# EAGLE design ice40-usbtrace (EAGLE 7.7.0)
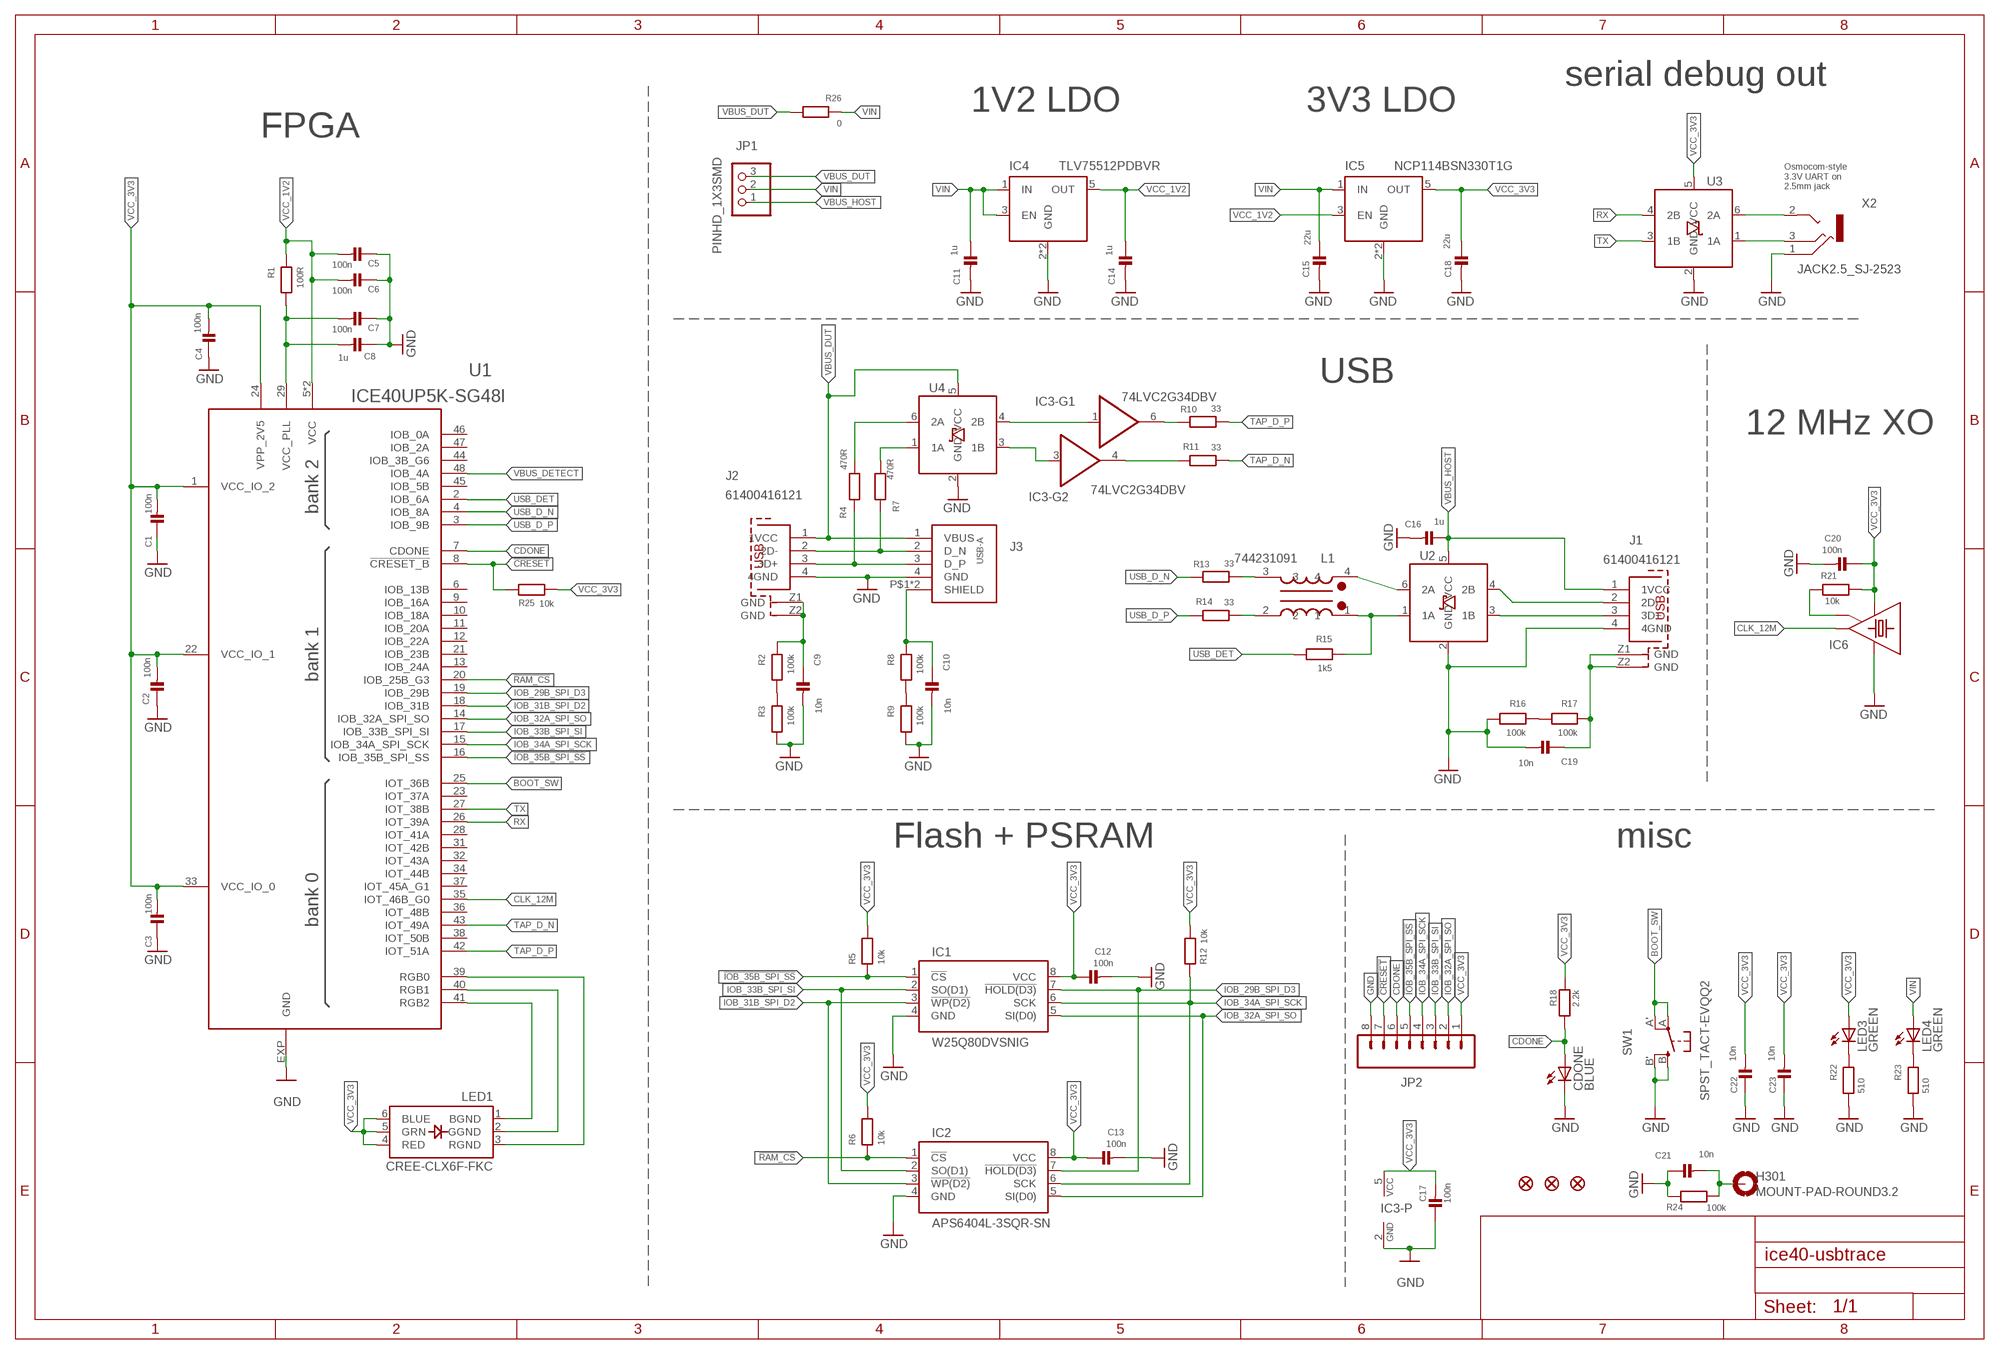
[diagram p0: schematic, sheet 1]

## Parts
C1  100n  CAP_CERAMIC_0603  [_0603]
C2  100n  CAP_CERAMIC_0603  [_0603]
C3  100n  CAP_CERAMIC_0603  [_0603]
C4  100n  CAP_CERAMIC_0603  [_0603]
C5  100n  CAP_CERAMIC_0603  [_0603]
C6  100n  CAP_CERAMIC_0603  [_0603]
C7  100n  CAP_CERAMIC_0603  [_0603]
C8  1u  CAP_CERAMIC_0603  [_0603]
C9  10n  CAP_CERAMIC_0402  [_0402]
C10  10n  CAP_CERAMIC_0402  [_0402]
C11  1u  CAP_CERAMIC_0603  [_0603]
C12  100n  CAP_CERAMIC_0603  [_0603]
C13  100n  CAP_CERAMIC_0603  [_0603]
C14  1u  CAP_CERAMIC_0603  [_0603]
C15  22u  CAP_CERAMIC1206  [1206]
C16  1u  CAP_CERAMIC_0603  [_0603]
C17  100n  CAP_CERAMIC_0603  [_0603]
C18  22u  CAP_CERAMIC1206  [1206]
C19  10n  CAP_CERAMIC_0402  [_0402]
C20  100n  CAP_CERAMIC_0603  [_0603]
C21  10n  CAP_CERAMIC_0402  [_0402]
C22  10n  CAP_CERAMIC_0402  [_0402]
C23  10n  CAP_CERAMIC_0402  [_0402]
CDONE  BLUE  LEDCHIPLED_0603  [CHIPLED_0603]
FID1  FIDUCIAL""  [FIDUCIAL_1MM]
FID2  FIDUCIAL""  [FIDUCIAL_1MM]
FID3  FIDUCIAL""  [FIDUCIAL_1MM]
H301  MOUNT-PAD-ROUND3.2  [3,2-PAD]
IC1  W25Q80DVSNIG  AT25SF-COMB  [SO08COMBINED]
IC2  APS6404L-3SQR-SN  AT25SF-COMB  [SO08COMBINED]
IC3  74LVC2G34DBV  [DBV_R-PDSO-G6]
IC4  TLV75512PDBVR  TLV70033-SOT  [SOT23-DBV]
IC5  NCP114BSN330T1G  TLV70033-SOT  [SOT23-DBV]
IC6  OSCILLATOR-4-SMD-2X2.5MM  [CRYSTAL-SMD-2X2.5MM]
J1  61400416121  [61400416121]
J2  61400416121  [61400416121]
J3  USB-A-HORIZ  [USB_A_HORIZ]
JP1  PINHD_1X3SMD  [1X03_SMD]
JP2  M08LOCK  [1X08_LOCK]
L1  744231091  WE-CNSW_0805  [WE-CNSW_0805]
LED1  CREE-CLX6F-FKC  [CREE-CLX6F-FKC_PLCC6]
LED3  GREEN  LEDCHIP-LED0603  [CHIP-LED0603]
LED4  GREEN  LEDCHIP-LED0603  [CHIP-LED0603]
R1  100R  RESISTOR_0603  [_0603]
R2  100k  RESISTOR_0603  [_0603]
R3  100k  RESISTOR_0603  [_0603]
R4  470R  RESISTOR_0603  [_0603]
R5  10k  RESISTOR_0603  [_0603]
R6  10k  RESISTOR_0603  [_0603]
R7  470R  RESISTOR_0603  [_0603]
R8  100k  RESISTOR_0603  [_0603]
R9  100k  RESISTOR_0603  [_0603]
R10  33  RESISTOR_0402  [_0402]
R11  33  RESISTOR_0402  [_0402]
R12  10k  RESISTOR_0603  [_0603]
R13  33  RESISTOR_0402  [_0402]
R14  33  RESISTOR_0402  [_0402]
R15  1k5  RESISTOR_0603  [_0603]
R16  100k  RESISTOR_0603  [_0603]
R17  100k  RESISTOR_0603  [_0603]
R18  2.2k  RESISTOR_0603  [_0603]
R21  10k  RESISTOR_0603  [_0603]
R22  510  RESISTOR_0603  [_0603]
R23  510  RESISTOR_0603  [_0603]
R24  100k  RESISTOR_0603  [_0603]
R25  10k  RESISTOR_0603  [_0603]
R26  0  RESISTOR_0603  [_0603]
SW1  SPST_TACT-EVQQ2  [EVQ-Q2]
U1  ICE40UP5K-SG48I  [QFN48]
U2  IP4234CZ6  [TSOP-6]
U3  IP4234CZ6  [TSOP-6]
U4  IP4234CZ6  [TSOP-6]
X2  JACK2.5_SJ-2523  [JACK2.5_SJ-2523]

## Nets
!CRESET: JP2.7 R25.1 U1.8(!CRESET_B)
!IOB_35B_SPI_SS: IC1.1(!CS) JP2.5 R5.1 U1.16(IOB_35B_SPI_SS)
!RAM_CS: IC2.1(!CS) R6.1 U1.20(IOB_25B_G3)
BOOT_SW: SW1.A'(P1) SW1.A(P) U1.25(IOT_36B)
CDONE: CDONE.A JP2.6 R18.2 U1.7(CDONE)
CLK_12M: IC6.3(OUT) U1.35(IOT_46B_G0)
GND [supply]: C1.1 C2.1 C3.1 C4.1 C5.1 C6.1 C7.1 C8.1 C9.2 C10.2 C11.2 C12.2 C13.2 C14.2 C15.2 C16.2 C17.1 C18.2 C19.2 C20.2 C21.1 C22.1 C23.1 CDONE.C IC1.4(GND) IC2.4(GND) IC3.2(-P:GND) IC4.2(GND) IC4.4(GND) IC5.2(GND) IC5.4(GND) IC6.2(GND) J1.4(4GND) J2.4(4GND) J3.4(GND) JP2.8 R3.1 R9.1 R16.1 R22.1 R23.1 R24.2 SW1.B'(S1) SW1.B(S) U1.EXP(GND) U2.2(GND) U3.2(GND) U4.2(GND) X2.1(RING)
IOB_29B_SPI_D3: IC1.7(!HOLD(D3)) IC2.7(!HOLD(D3)) U1.19(IOB_29B)
IOB_31B_SPI_D2: IC1.3(!WP(D2)) IC2.3(!WP(D2)) U1.18(IOB_31B)
IOB_32A_SPI_SO: IC1.5(SI(D0)) IC2.5(SI(D0)) JP2.2 U1.14(IOB_32A_SPI_SO)
IOB_33B_SPI_SI: IC1.2(SO(D1)) IC2.2(SO(D1)) JP2.3 U1.17(IOB_33B_SPI_SI)
IOB_34A_SPI_SCK: IC1.6(SCK) IC2.6(SCK) JP2.4 R12.1 U1.15(IOB_34A_SPI_SCK)
N$1: LED1.2(GGND) U1.40(RGB1)
N$2: U3.6(2A) X2.2(TIP)
N$3: R7.2 U4.1(1A)
N$3_N [usb]: J2.2(2D-) J3.2(D_N) R7.1
N$3_P [usb]: J2.3(3D+) J3.3(D_P) R4.1
N$4: C21.2 H301.B3,2(MOUNT) R24.1
N$5: LED3.C R22.2
N$6: R2.1 R3.2
N$7: R8.1 R9.2
N$8: R4.2 U4.6(2A)
N$9: C10.1 J3.P$1(SHIELD) J3.P$2(SHIELD) R8.2
N$10: IC3.1(-G1:A) U4.4(2B)
N$11: C9.1 J2.Z1(GND) J2.Z2(GND) R2.2
N$12: IC3.4(-G2:Y) R11.1
N$13: IC3.6(-G1:Y) R10.1
N$14: LED4.C R23.2
N$15: IC3.3(-G2:A) U4.3(1B)
N$17_D_N [usb]: L1.3 R13.2
N$17_D_P [usb]: L1.2 R14.2
N$25: IC6.1(EN) R21.1
N$45: LED1.1(BGND) U1.41(RGB2)
N$52: C7.2 C8.2 R1.1 U1.29(VCC_PLL)
N$55: R16.2 R17.1
N$61: C19.1 J1.Z1(GND) J1.Z2(GND) R17.2
N$63: LED1.3(RGND) U1.39(RGB0)
RX: U1.26(IOT_39A) U3.4(2B)
TAP_D_N [usb]: R11.2 U1.43(IOT_49A)
TAP_D_P [usb]: R10.2 U1.42(IOT_51A)
TX: U1.27(IOT_38B) U3.3(1B)
UART_TX0: U3.1(1A) X2.3(MIDDLE)
USB0_D_N [usb]: J1.2(2D-) U2.4(2B)
USB0_D_P [usb]: J1.3(3D+) U2.3(1B)
USB1_D_N [usb]: L1.4 U2.6(2A)
USB1_D_P [usb]: L1.1 R15.2 U2.1(1A)
USB_D_N [usb]: R13.1 U1.4(IOB_8A)
USB_D_P [usb]: R14.1 U1.3(IOB_9B)
USB_DET: R15.1 U1.2(IOB_6A)
VBUS_DETECT: U1.48(IOB_4A)
VBUS_DUT [supply]: J2.1(1VCC) J3.1(VBUS) JP1.3 R26.1 U4.5(VCC)
VBUS_HOST [supply]: C16.1 J1.1(1VCC) JP1.1 U2.5(VCC)
VCC_1V2 [supply]: C5.2 C6.2 C14.1 IC4.5(OUT) IC5.3(EN) R1.2 U1.5(VCC) U1.30(VCC)
VCC_3V3 [supply]: C1.2 C2.2 C3.2 C4.2 C12.1 C13.1 C17.2 C18.1 C20.1 C22.2 C23.2 IC1.8(VCC) IC2.8(VCC) IC3.5(-P:VCC) IC5.5(OUT) IC6.4(VCC) JP2.1 LED1.4(RED) LED1.5(GRN) LED1.6(BLUE) LED3.A R5.2 R6.2 R12.2 R18.1 R21.2 R25.2 U1.1(VCC_IO_2) U1.22(VCC_IO_1) U1.24(VPP_2V5) U1.33(VCC_IO_0) U3.5(VCC)
VIN [supply]: C11.1 C15.1 IC4.1(IN) IC4.3(EN) IC5.1(IN) JP1.2 LED4.A R26.2
Unconnected: U1.6(IOB_13B) U1.9(IOB_16A) U1.10(IOB_18A) U1.11(IOB_20A) U1.12(IOB_22A) U1.13(IOB_24A) U1.21(IOB_23B) U1.23(IOT_37A) U1.28(IOT_41A) U1.31(IOT_42B) U1.32(IOT_43A) U1.34(IOT_44B) U1.36(IOT_48B) U1.37(IOT_45A_G1) U1.38(IOT_50B) U1.44(IOB_3B_G6) U1.45(IOB_5B) U1.46(IOB_0A) U1.47(IOB_2A)

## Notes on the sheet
- serial debug out
- 1V2 LDO | 3V3 LDO
- FPGA
- Osmocom-style
  3.3V UART on
  2.5mm jack
- USB
- 12 MHz XO
- Flash + PSRAM | misc

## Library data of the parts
C1-C7 C12 C13 C17 C20 = rc-sysmocom:CAP_CERAMIC: Ceramic Capacitors; CLASS: CAPACITOR; DESCRIPTION: CAP CER 0.1UF 16V 10% X7R 0603; LINK: http://www.digikey.de/product-detail/de/foo/1276-1005-1-ND; MANUFACTURER: Samsung Electro-Mechanics America, Inc; MANUFACTURERPARTNUMBER: CL10B104KO8NNNC; POPULATED: TRUE; ROHSCERTIFICATE: Bleifrei / RoHS-konform; SOURCE: DIGIKEY; SOURCEPARTNUMBER: 1276-1005-1-ND
C8 C11 C14 C16 = rc-sysmocom:CAP_CERAMIC: Ceramic Capacitors; CLASS: CAPACITOR; DESCRIPTION: CAP CER 1UF 10V X5R 0603; LINK: https://www.digikey.de/product-detail/de/samsung-electro-mechanics/CL10A105KP8NNNC/1276-1182-1-ND/3889268; MANUFACTURER: Samsung Electro-Mechanics; MANUFACTURERPARTNUMBER: CL10A105KP8NNNC; POPULATED: TRUE; ROHSCERTIFICATE: Bleifrei / RoHS-konform; SOURCE: DIGIKEY; SOURCEPARTNUMBER: 1276-1182-1-ND
C9 C10 C19 C21-C23 = rc-sysmocom:CAP_CERAMIC: Ceramic Capacitors; CLASS: CAPACITOR; DESCRIPTION: CAP CER 10000PF 25V X7R 0402; LINK: https://www.digikey.de/product-detail/de/samsung-electro-mechanics/CL05B103KA5NNNC/1276-1057-1-ND/3889143; MANUFACTURER: Samsung Electro-Mechanics; MANUFACTURERPARTNUMBER: CL05B103KA5NNNC; POPULATED: TRUE; ROHSCERTIFICATE: Bleifrei / RoHS-konform; SOURCE: DIGIKEY; SOURCEPARTNUMBER: 1276-1057-1-ND
C15 C18 = rc-sysmocom:CAP_CERAMIC: Ceramic Capacitors; CLASS: CAPACITOR; DESCRIPTION: CAP CER 22UF 10V 10% X5R 1206; LINK: http://www.digikey.de/product-detail/de/foo/1276-1287-1-ND; MANUFACTURER: Samsung Electro-Mechanics America, Inc; MANUFACTURERPARTNUMBER: CL31A226KPHNNNE; POPULATED: TRUE; ROHSCERTIFICATE: Bleifrei / RoHS-konform; SOURCE: DIGIKEY; SOURCEPARTNUMBER: 1276-1287-1-ND
CDONE = led:LED: LED; CLASS: LED; DESCRIPTION: LED BLUE CLEAR CHIP SMD; LINK: https://www.digikey.de/de/products/detail/liteon/LTST-C193TBKT-5A/2053656; MANUFACTURER: Lite-On Inc.; MANUFACTURERPARTNUMBER: LTST-C193TBKT-5A; POPULATED: TRUE; ROHSCERTIFICATE: RoHS3-konform; SOURCE: DIGIKEY; SOURCEPARTNUMBER: 160-1827-1-ND
FID1-FID3 = microbuilder:FIDUCIAL: Fiducial Alignment Points; CLASS: UNKNOWN CLASS; DESCRIPTION: NO DESCRIPTION; LINK: UNKNOWN LINK; MANUFACTURER: UNKNOWN MANUFACTURER; MANUFACTURERPARTNUMBER: UNKNOWN MANUFACTURER PART NUMBER; POPULATED: TRUE; ROHSCERTIFICATE: UNKNOWN ROHS CERTIFICATE; SOURCE: UNKNOWN SOURCE; SOURCEPARTNUMBER: UNKNOWN SOURCE PART NUMBER
H301 = holes:MOUNT-PAD-ROUND: MOUNTING PAD, round; CLASS: HOLE; DESCRIPTION: NO DESCRIPTION; LINK: UNKNOWN LINK; MANUFACTURER: UNKNOWN MANUFACTURER; MANUFACTURERPARTNUMBER: UNKNOWN MANUFACTURER PART NUMBER; POPULATED: FALSE; ROHSCERTIFICATE: UNKNOWN ROHS CERTIFICATE; SOURCE: UNKNOWN SOURCE; SOURCEPARTNUMBER: UNKNOWN SOURCE PART NUMBER
IC1 = spiflash:AT25SF; CLASS: IC; DESCRIPTION: IC FLASH 8M SPI 104MHZ 8SOIC; LINK: https://www.digikey.de/de/products/detail/winbond-electronics/W25Q80DVSNIG/4878496; MANUFACTURER: Winbond Electronics; MANUFACTURERPARTNUMBER: W25Q80DVSNIG; POPULATED: TRUE; ROHSCERTIFICATE: RoHS3-konform; SOURCE: DIGIKEY; SOURCEPARTNUMBER: W25Q80DVSNIG-ND
IC2 = spiflash:AT25SF; CLASS: IC; DESCRIPTION: PSRAM 64Mb QSPI (x1,x4) 133/84MHz SOIC8; LINK: https://www.mouser.de/ProductDetail/AP-Memory/APS6404L-3SQR-SN?qs=IS%252B4QmGtzzqsn3S5xo%2FEEg%3D%3D; MANUFACTURER: AP Memory; MANUFACTURERPARTNUMBER: APS6404L-3SQR-SN; POPULATED: TRUE; ROHSCERTIFICATE: UNKNOWN ROHS CERTIFICATE; SOURCE: MOUSER; SOURCEPARTNUMBER: 878-APS6404L-3SQR-SN
IC3 = 74LVC2G34:74LVC2G34: Dual Buffer/Driver with open drain output; CLASS: IC; DESCRIPTION: IC BUF NON-INVERT 5.5V SOT23-6; LINK: https://www.digikey.de/de/products/detail/texas-instruments/SN74LVC2G34DBVT/2261911; MANUFACTURER: TI; MANUFACTURERPARTNUMBER: SN74LVC2G34DBVT; POPULATED: TRUE; ROHSCERTIFICATE: UNKNOWN ROHS CERTIFICATE; SOURCE: DIGIKEY; SOURCEPARTNUMBER: 296-32325-6-ND
IC4 = tlv700xx:TLV700*: TLV700xx also works for SOT variants of TLV702xx and TLV733xx; CLASS: IC; DESCRIPTION: IC REG LINEAR 1.2V 500MA SOT23-5; LINK: https://www.digikey.de/de/products/detail/texas-instruments/TLV75512PDBVR/9356525; MANUFACTURER: UNKNOWN MANUFACTURER; MANUFACTURERPARTNUMBER: TLV75512PDBVR; POPULATED: TRUE; ROHSCERTIFICATE: UNKNOWN ROHS CERTIFICATE; SOURCE: DIGIKEY; SOURCEPARTNUMBER: 296-50409-1-ND
IC5 = tlv700xx:TLV700*: TLV700xx also works for SOT variants of TLV702xx and TLV733xx; CLASS: IC; DESCRIPTION: IC REG LINEAR 3.3V 300MA 5TSOP; LINK: https://www.digikey.de/de/products/detail/onsemi/NCP114BSN330T1G/6560606; MANUFACTURER: UNKNOWN MANUFACTURER; MANUFACTURERPARTNUMBER: NCP114BSN330T1G; POPULATED: TRUE; ROHSCERTIFICATE: UNKNOWN ROHS CERTIFICATE; SOURCE: DIGIKEY; SOURCEPARTNUMBER: NCP114BSN330T1GOSCT-ND
IC6 = XO-2x2.5mm:OSCILLATOR-4: 4pin-oscillator, 2.5 x 2mm; CLASS: XTAL / OSCILLATOR; DESCRIPTION: XTAL OSC XO 12MHZ HCMOS SMD; LINK: https://www.digikey.de/de/products/detail/jauch-quartz/O-12-0-JO22-B-1V3-1-T1-LF/10416129; MANUFACTURER: Jauch Quartz; MANUFACTURERPARTNUMBER: O 12,0-JO22-B-1V3-1-T1-LF; POPULATED: TRUE; ROHSCERTIFICATE: UNKNOWN ROHS CERTIFICATE; SOURCE: DIGIKEY; SOURCEPARTNUMBER: 1908-O120-JO22-B-1V3-1-T1-LFCT-ND
J1 J2 = Wuerth_Elektronik_eiCan_Communication_Connectors_v6_20150113:61400416121: WR-COM Horizontal USB Type B=>Code : Con_I-O_COM_USB-2.0_B_61400416121 Details see: http://katalog.we-online.de/en/em/614_004_161_21 Created 2014-07-09, Karrer Zheng 2014 (C) Würth Elektronik; CLASS: CONNECTOR; DESCRIPTION: CONN RCPT USB2.0 TYPEB 4POS R/A; LINK: https://www.digikey.de/product-detail/de/wurth-electronics-inc/61400416121/732-2108-ND; MANUFACTURER: Würth Elektronik; MANUFACTURERPARTNUMBER: 61400416121; POPULATED: TRUE; ROHSCERTIFICATE: UNKNOWN ROHS CERTIFICATE; SOURCE: DIGIKEY; SOURCEPARTNUMBER: 732-2108-ND
J3 = laforge:USB-A: USB A socket THT Amphenol UE27-AEX4-X0X; CLASS: CONNECTOR; DESCRIPTION: CONN RCPT USB2.0 TYPEA 4POS R/A; LINK: https://www.digikey.de/product-detail/de/wurth-electronics-inc/61400416021/732-2106-ND; MANUFACTURER: Würth Elektronik; MANUFACTURERPARTNUMBER: 61400416021; POPULATED: TRUE; ROHSCERTIFICATE: UNKNOWN ROHS CERTIFICATE; SOURCE: DIGIKEY; SOURCEPARTNUMBER: 732-2106-ND
JP1 = laforge:PINHD_1X3; CLASS: CONNECTOR\JUMPER; DESCRIPTION: NO DESCRIPTION; LINK: UNKNOWN LINK; MANUFACTURER: UNKNOWN MANUFACTURER; MANUFACTURERPARTNUMBER: UNKNOWN MANUFACTURER PART NUMBER; POPULATED: FALSE; ROHSCERTIFICATE: UNKNOWN ROHS CERTIFICATE; SOURCE: UNKNOWN SOURCE; SOURCEPARTNUMBER: UNKNOWN SOURCE PART NUMBER
JP2 = SparkFun-Connectors:M08: Header 8 Standard 8-pin 0.1" header. Use with straight break away headers (SKU : PRT-00116), right angle break away headers (PRT-00553), swiss pins (PRT-00743), machine pins (PRT-00117), and female headers (PRT-00115).; CLASS: CONNECTOR\JUMPER; DESCRIPTION: NO DESCRIPTION; LINK: UNKNOWN LINK; MANUFACTURER: UNKNOWN MANUFACTURER; MANUFACTURERPARTNUMBER: UNKNOWN MANUFACTURER PART NUMBER; POPULATED: FALSE; ROHSCERTIFICATE: UNKNOWN ROHS CERTIFICATE; SOURCE: UNKNOWN SOURCE; SOURCEPARTNUMBER: UNKNOWN SOURCE PART NUMBER
L1 = Wuerth_Elektronik_eiSos_V6_20140807:WE-CNSW: SMD Common Mode Noise Suppressor WE-CNSW - High common mode suppression at high frequency - Small influence for high speed signals through winding symmetry -- USB 2.0 -- Firewire / IEEE 1394 -- Power supply systems -- High Speed Data Lines -- Common mode data line filter Details see: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; CLASS: INDUCTOR; DESCRIPTION: CMC 370MA 2LN 90 OHM SMD; LINK: https://www.digikey.de/product-detail/de/wurth-electronics-inc/744231091/732-3198-1-ND; MANUFACTURER: Wurth Electronics Inc.; MANUFACTURERPARTNUMBER: 744231091; POPULATED: TRUE; ROHSCERTIFICATE: Bleifrei / RoHS-konform; SOURCE: DIGIKEY; SOURCEPARTNUMBER: 732-3198-1-ND
LED1 = CREE_CLX6F-FKC:CREE-CLX6F-FKC: Cree CLX6F-FKC PLCC6 3 in 1 SMD LED 1mm pitch; CLASS: LED; DESCRIPTION: NO DESCRIPTION; LINK: https://www.digikey.de/de/products/detail/creeled-inc/CLX6F-FKC-CKNNQDGBB7A363/6355679; MANUFACTURER: CreeLED, Inc; MANUFACTURERPARTNUMBER: CLX6F-FKC-CKNNQDGBB7A363; POPULATED: TRUE; ROHSCERTIFICATE: UNKNOWN ROHS CERTIFICATE; SOURCE: DIGIKEY; SOURCEPARTNUMBER: CLX6F-FKC-CKNNQDGBB7A363DKR-ND
LED3 LED4 = led:LED: LED; CLASS: LED; DESCRIPTION: NO DESCRIPTION; LINK: UNKNOWN LINK; MANUFACTURER: UNKNOWN MANUFACTURER; MANUFACTURERPARTNUMBER: UNKNOWN MANUFACTURER PART NUMBER; POPULATED: TRUE; ROHSCERTIFICATE: UNKNOWN ROHS CERTIFICATE; SOURCE: UNKNOWN SOURCE; SOURCEPARTNUMBER: UNKNOWN SOURCE PART NUMBER
R1 = rc-sysmocom:RESISTOR: Resistors; CLASS: RESISTOR; DESCRIPTION: RES 100 OHM 5%% 1/10W 0603; LINK: https://www.digikey.de/product-detail/de/stackpole-electronics-inc/RMCF0603JT100R/RMCF0603JT100RCT-ND; MANUFACTURER: Stackpole Electronics Inc; MANUFACTURERPARTNUMBER: RMCF0603JT100R; POPULATED: TRUE; ROHSCERTIFICATE: RoHS3-konform; SOURCE: DIGIKEY; SOURCEPARTNUMBER: RMCF0603JT100RCT-ND
R2 R3 R8 R9 R16 R17 R24 = rc-sysmocom:RESISTOR: Resistors; CLASS: RESISTOR; DESCRIPTION: RES SMD 100K OHM 5%% 1/10W 0603; LINK: https://www.digikey.de/product-detail/de/yageo/RC0603JR-07100KL/311-100KGRCT-ND/729645; MANUFACTURER: Yageo; MANUFACTURERPARTNUMBER: RC0603JR-07100KL; POPULATED: TRUE; ROHSCERTIFICATE: Bleifrei / RoHS-konform; SOURCE: DIGIKEY; SOURCEPARTNUMBER: 311-100KGRCT-ND
R4 R7 = rc-sysmocom:RESISTOR: Resistors; CLASS: RESISTOR; DESCRIPTION: RES 470 OHM 1% 1/10W 0603; LINK: https://www.digikey.de/de/products/detail/stackpole-electronics-inc/RMCF0603FT470R/1761144; MANUFACTURER: Stackpole Electronics Inc; MANUFACTURERPARTNUMBER: RMCF0603FT470R; POPULATED: TRUE; ROHSCERTIFICATE: UNKNOWN ROHS CERTIFICATE; SOURCE: DIGIKEY; SOURCEPARTNUMBER: RMCF0603FT470RCT-ND
R5 R6 R12 R21 R25 = rc-sysmocom:RESISTOR: Resistors; CLASS: RESISTOR; DESCRIPTION: RES 10K OHM 5%% 1/10W 0603; LINK: https://www.digikey.de/product-detail/de/stackpole-electronics-inc/RMCF0603JT10K0/RMCF0603JT10K0CT-ND; MANUFACTURER: Stackpole Electronics Inc; MANUFACTURERPARTNUMBER: RMCF0603JT10K0; POPULATED: TRUE; ROHSCERTIFICATE: RoHS3-konform; SOURCE: DIGIKEY; SOURCEPARTNUMBER: RMCF0603JT10K0CT-ND
R10 R11 R13 R14 = rc-sysmocom:RESISTOR: Resistors; CLASS: RESISTOR; DESCRIPTION: RES SMD 33 OHM 1%% 1/16W 0402; LINK: https://www.digikey.de/product-detail/de/yageo/RC0402FR-0733RL/311-33-0LRCT-ND/729540; MANUFACTURER: Yageo; MANUFACTURERPARTNUMBER: RC0402FR-0733RL; POPULATED: TRUE; ROHSCERTIFICATE: RoHS3-konform; SOURCE: DIGIKEY; SOURCEPARTNUMBER: 311-33.0LRCT-ND
R15 = rc-sysmocom:RESISTOR: Resistors; CLASS: RESISTOR; DESCRIPTION: RES 1.5K OHM 5%% 1/10W 0603; LINK: https://www.digikey.de/product-detail/de/stackpole-electronics-inc/RMCF0603JT1K50/RMCF0603JT1K50CT-ND; MANUFACTURER: Stackpole Electronics Inc; MANUFACTURERPARTNUMBER: RMCF0603JT1K50; POPULATED: TRUE; ROHSCERTIFICATE: RoHS3-konform; SOURCE: DIGIKEY; SOURCEPARTNUMBER: RMCF0603JT1K50CT-ND
R18 = rc-sysmocom:RESISTOR: Resistors; CLASS: RESISTOR; DESCRIPTION: RES 2.2K OHM 5%% 1/10W 0603; LINK: https://www.digikey.de/product-detail/de/stackpole-electronics-inc/RMCF0603JT2K20/RMCF0603JT2K20CT-ND; MANUFACTURER: Stackpole Electronics Inc; MANUFACTURERPARTNUMBER: RMCF0603JT2K20; POPULATED: TRUE; ROHSCERTIFICATE: RoHS3-konform; SOURCE: DIGIKEY; SOURCEPARTNUMBER: RMCF0603JT2K20CT-ND
R22 R23 = rc-sysmocom:RESISTOR: Resistors; CLASS: RESISTOR; DESCRIPTION: RES 510 OHM 1%% 1/10W 0603; LINK: https://www.digikey.de/product-detail/de/stackpole-electronics-inc/RMCF0603FT510R/RMCF0603FT510RCT-ND; MANUFACTURER: Stackpole Electronics Inc; MANUFACTURERPARTNUMBER: RMCF0603FT510R; POPULATED: TRUE; ROHSCERTIFICATE: RoHS3-konform; SOURCE: DIGIKEY; SOURCEPARTNUMBER: RMCF0603FT510RCT-ND
R26 = rc-sysmocom:RESISTOR: Resistors; CLASS: RESISTOR; DESCRIPTION: RES SMD 0 OHM JUMPER 1/10W 0603; LINK: https://www.digikey.de/product-detail/de/yageo/RC0603JR-070RL/311-0.0GRCT-ND; MANUFACTURER: Yageo; MANUFACTURERPARTNUMBER: RC0603JR-070RL; POPULATED: TRUE; ROHSCERTIFICATE: Bleifrei / RoHS-konform; SOURCE: DIGIKEY; SOURCEPARTNUMBER: 311-0.0GRCT-ND
SW1 = adafruit:SPST_TACT: SMT 6mm switch, EVQQ2 series http://www.ladyada.net/library/eagle; CLASS: SWITCH; DESCRIPTION: SWITCH TACTILE SPST-NO 0.02A 15V; LINK: https://www.digikey.de/de/products/detail/panasonic-electronic-components/EVQ-Q2B03W/762882; MANUFACTURER: Panasonic Electronic Components; MANUFACTURERPARTNUMBER: EVQ-Q2B03W; POPULATED: TRUE; ROHSCERTIFICATE: UNKNOWN ROHS CERTIFICATE; SOURCE: DIGIKEY; SOURCEPARTNUMBER: P12932SCT-ND
U1 = ice40:ICE40UP5K-SG48I: Field Programmable Gate Array iCE40-UltraPlus, 5280 LUTs, 1.2V; CLASS: IC; DESCRIPTION: IC FPGA 39 I/O 48QFN; LINK: https://www.digikey.de/product-detail/de/lattice-semiconductor-corporation/ICE40UP5K-SG48I/220-2212-1-ND/; MANUFACTURER: Lattice Semiconductor Corporation; MANUFACTURERPARTNUMBER: ICE40UP5K-SG48I; POPULATED: TRUE; ROHSCERTIFICATE: RoHS3-konform; SOURCE: DIGIKEY; SOURCEPARTNUMBER: 220-2212-1-ND
U2 U4 = laforge:IP4234CZ6: NXP IP4234CZ6 - Single USB 2.0 ESD protection to IEC 61000-4-2 level 4; CLASS: IC; DESCRIPTION: TVS DIODE 5.5V 6TSOP; LINK: https://www.digikey.de/product-detail/de/nexperia-usa-inc/IP4234CZ6125/1727-4717-1-ND/2531156; MANUFACTURER: Nexperia USA Inc.; MANUFACTURERPARTNUMBER: IP4234CZ6,125; OC_DIGIKEY: 568-5869-1-ND; POPULATED: TRUE; ROHSCERTIFICATE: Bleifrei / RoHS-konform; SOURCE: DIGIKEY; SOURCEPARTNUMBER: 1727-4717-1-ND
U3 = laforge:IP4234CZ6: NXP IP4234CZ6 - Single USB 2.0 ESD protection to IEC 61000-4-2 level 4; CLASS: IC; DESCRIPTION: TVS DIODE 5.5V 6TSOP; LINK: https://www.digikey.de/product-detail/de/nexperia-usa-inc/IP4234CZ6125/1727-4717-1-ND/2531156; MANUFACTURER: Nexperia USA Inc.; MANUFACTURERPARTNUMBER: IP4234CZ6,125; OC_DIGIKEY: 568-5869-1-ND; POPULATED: FALSE; ROHSCERTIFICATE: Bleifrei / RoHS-konform; SOURCE: DIGIKEY; SOURCEPARTNUMBER: 1727-4717-1-ND
X2 = laforge:JACK2.5_SJ-2523: CUI Inc. SJ-2523-SMT; CLASS: CONNECTOR; DESCRIPTION: CONN JACK STEREO 2.5MM SMD R/A; LINK: https://www.digikey.de/product-detail/de/cui-inc/SJ-2523-SMT-TR/CP-2523SJCT-ND/669702; MANUFACTURER: CUI Inc.; MANUFACTURERPARTNUMBER: SJ-2523-SMT-TR; OC_DIGIKEY: CP-2523SJCT-ND; POPULATED: FALSE; ROHSCERTIFICATE: Bleifrei / RoHS-konform; SOURCE: DIGIKEY; SOURCEPARTNUMBER: CP-2523SJCT-ND

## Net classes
0 default: width 0.3 mm
1 usb: width 0.7 mm, clearance 0.15 mm
2 fgt: width 0.6 mm, drill 0.2 mm, clearance 0.2 mm to class 0, clearance 0.2 mm to class 1, clearance 0.2 mm
3 supply: width 0.6 mm, clearance 0.3 mm to class 0, clearance 0.3 mm to class 1, clearance 0.3 mm to class 2, clearance 0.3 mm

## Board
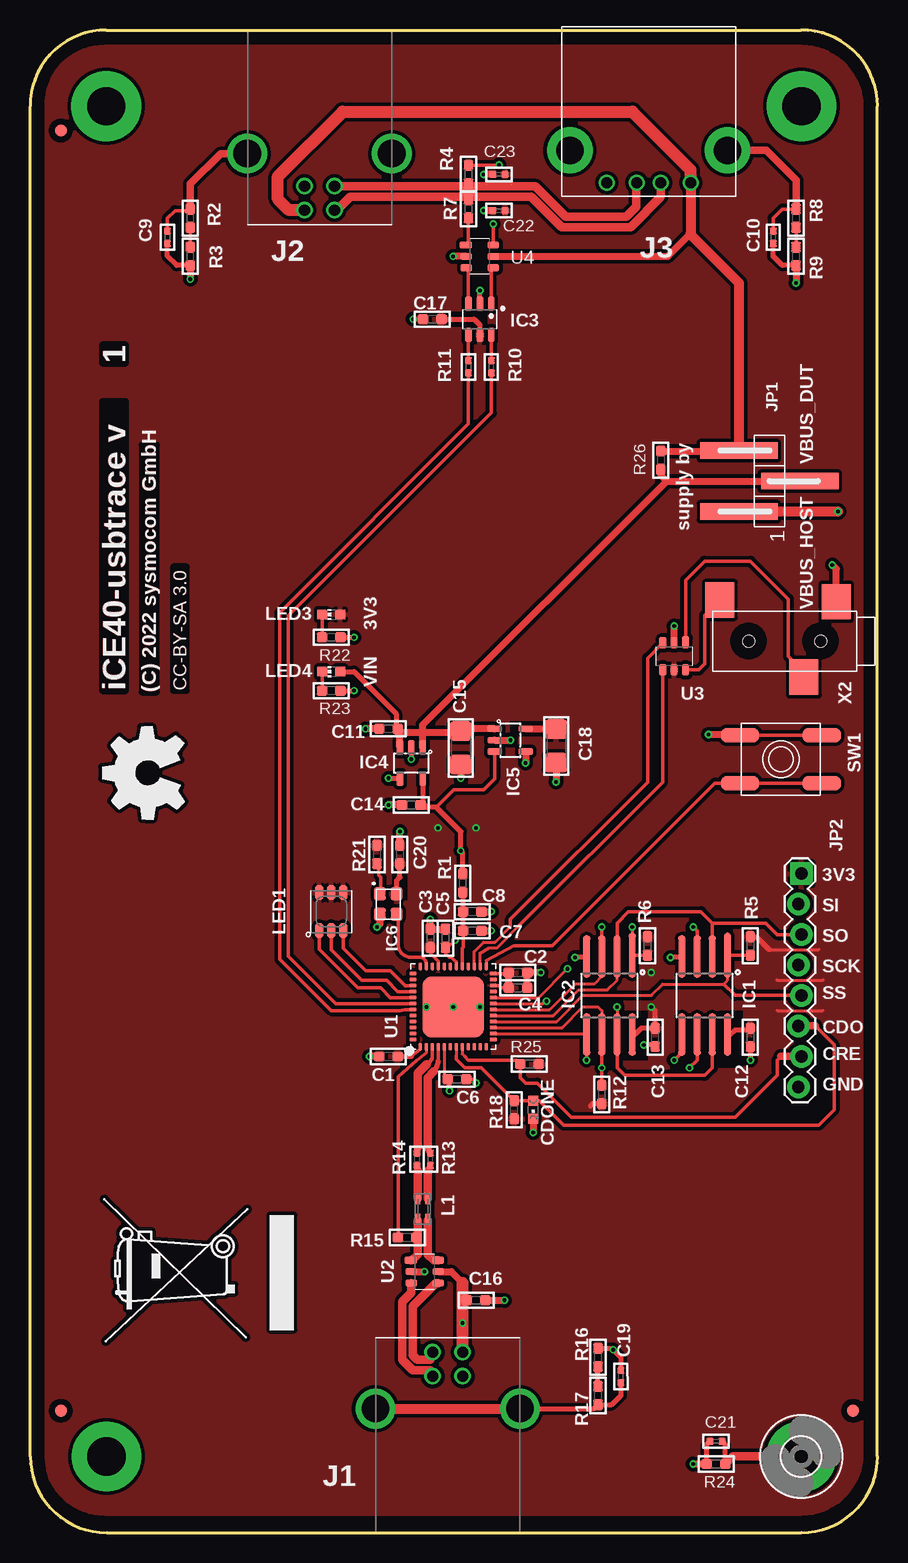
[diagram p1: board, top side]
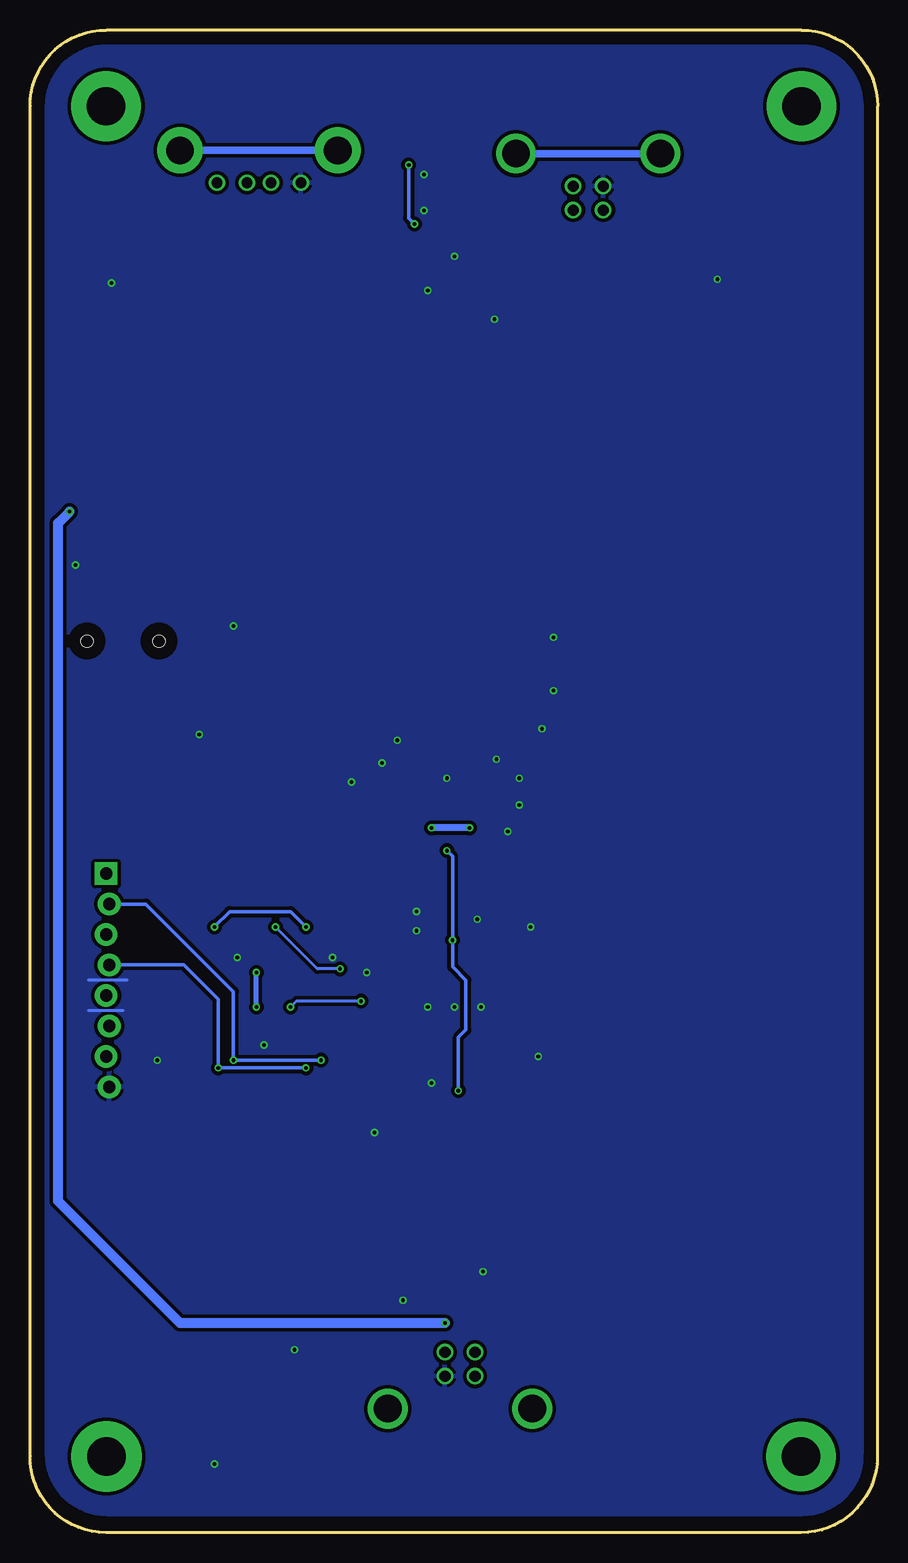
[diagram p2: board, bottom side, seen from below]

Size 70.64 x 125.22 mm. Coordinates in mm from the lower left corner, seen from the top.
Outline: 70.64,118.87 arc90 64.26,125.22
Outline: 0,118.85 arc-90 6.35,125.22 64.26,125.22
Outline: 0.02,6.35 arc90 6.4,0
Outline: 70.64,6.37 arc-90 64.29,0 6.4,0
Outline: 70.61,6.38 70.61,118.87
Outline: 0,6.35 0,118.85
Copper layers (1*16): Top 0.035mm / dielectric 1.5mm / Bottom 0.035mm
Design rules "sysmocom-def *": minimum track width 4mil, minimum drill 0.3mm, track to track 6mil, track to pad 6mil, pad to pad 6mil, via to via 6mil, smd to smd 0mil, copper to edge 40mil, drill to drill 8mil, minimum pad ring 6mil, minimum via ring 6mil, stop-mask expansion 4mil, vias tented up to drill 0mil, thermal gap 10mil
tRestrict: area 57.5,38.7 to 59.4,43.5; area 34.9,100.5 to 38.1,101.8; area 38.4,46.7 to 39.4,47.3; area 39.1,45.1 to 39.7,45.7; area 30.2,52.7 to 31.5,55.2; area 31.8,26.4 to 33.7,27.6; area 32.7,47.6 to 34.6,48.3; area 40,66.4 to 43.8,67.6; area 31.1,38.4 to 33,40.6; area 49.6,39.4 to 51.5,43.5

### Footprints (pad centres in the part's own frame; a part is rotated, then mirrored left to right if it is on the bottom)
_0603 = smd 0.9 x 0.8: 1 -0.762,0; 2 0.762,0
_0402 = smd 0.6 x 0.6: 1 -0.508,0; 2 0.508,0
1206 = smd 1.6 x 1.8: 1 -1.4,0; 2 1.4,0
CHIPLED_0603 = smd 0.8 x 0.8: A 0,-0.75; C 0,0.75
FIDUCIAL_1MM = smd 1 x 1: 1 0,0
MOUNTING_HOLE_1PRIMARY = drill 3.2 pad 5.8: 1 0,0
MOUNTING_HOLE_2PRIMARY = drill 3.2 pad 5.8: 1 0.025,0
3,2-PAD = drill 3.2 pad 5.842: B3,2 0,0
SO08COMBINED = smd 0.6 x 3.7: 1 -1.905,-3.351 | smd 0.6 x 3.5: 2 -0.635,-3.251; 3 0.635,-3.251; 4 1.905,-3.251; 5 1.905,3.251; 6 0.635,3.251; 7 -0.635,3.251; 8 -1.905,3.251
DBV_R-PDSO-G6 = smd 0.55 x 1.2: 1 -0.95,-1.3; 2 0,-1.3; 3 0.95,-1.3; 4 0.95,1.3; 5 0,1.3; 6 -0.95,1.3
SOT23-DBV = smd 0.55 x 1.2: 1 -0.95,-1.3; 2 0,-1.3; 3 0.95,-1.3; 4 0.95,1.3; 5 -0.95,1.3
CRYSTAL-SMD-2X2.5MM = smd 1.1 x 1: 1 -0.854,-0.71; 2 0.846,-0.71; 3 0.846,0.69; 4 -0.854,0.69
61400416121 = drill 0.92: 1 1.25,4.71; 2 -1.25,4.71; 3 -1.25,2.71; 4 1.25,2.71 | drill 2.3: Z1 -6.02,0; Z2 6.02,0
USB_A_HORIZ = drill 0.9: 1 -3.5,2.7; 2 -1,2.7; 3 1,2.7; 4 3.5,2.7 | drill 2.3 pad 3.81: P$1 -6.57,0; P$2 6.57,0
1X03_SMD = smd 1.37 x 6.45: 1 -2.54,2.54; 2 0,-2.54; 3 2.54,2.54
1X08_LOCK = drill 1.016 pad 1.88 square: 1 0,0.127 | drill 1.016 pad 1.88: 2 2.54,-0.127; 3 5.08,0.127; 4 7.62,-0.127; 5 10.16,0.127; 6 12.7,-0.127; 7 15.24,0.127; 8 17.78,-0.127
WE-CNSW_0805 = smd 0.4 x 0.9: 1 -0.4,-0.85; 2 -0.4,0.85; 3 0.4,0.85; 4 0.4,-0.85
CREE-CLX6F-FKC_PLCC6 = smd 1.27 x 0.7: 1 -1.587,1; 2 -1.587,0; 3 -1.587,-1; 4 1.587,-1; 5 1.587,0; 6 1.587,1
CHIP-LED0603 = smd 0.8 x 0.8: A 0,-0.75; C 0,0.75
EVQ-Q2 = smd 3.2 x 1.2: A -3.4,-2; A' 3.4,-2; B -3.4,2; B' 3.4,2
QFN48 = smd 0.6 x 0.3: 1 -3.32,2.75; 2 -3.32,2.25; 3 -3.32,1.75; 4 -3.32,1.25; 5 -3.32,0.75; 6 -3.32,0.25; 7 -3.32,-0.25; 8 -3.32,-0.75; 9 -3.32,-1.25; 10 -3.32,-1.75; 11 -3.32,-2.25; 12 -3.32,-2.75; 25 3.38,-2.75; 26 3.38,-2.25; 27 3.38,-1.75; 28 3.38,-1.25; 29 3.38,-0.75; 30 3.38,-0.25; 31 3.38,0.25; 32 3.38,0.75; 33 3.38,1.25; 34 3.38,1.75; 35 3.38,2.25; 36 3.38,2.75 | smd 0.3 x 0.6: 13 -2.72,-3.35; 14 -2.22,-3.35; 15 -1.72,-3.35; 16 -1.22,-3.35; 17 -0.72,-3.35; 18 -0.22,-3.35; 19 0.28,-3.35; 20 0.78,-3.35; 21 1.28,-3.35; 22 1.78,-3.35; 23 2.28,-3.35; 24 2.78,-3.35; 37 2.78,3.35; 38 2.28,3.35; 39 1.78,3.35; 40 1.28,3.35; 41 0.78,3.35; 42 0.28,3.35; 43 -0.22,3.35; 44 -0.72,3.35; 45 -1.22,3.35; 46 -1.72,3.35; 47 -2.22,3.35; 48 -2.72,3.35 | smd 5.08 x 5.08: EXP 0,0
TSOP-6 = smd 0.6 x 1.05: 1 -0.95,-1.175 | smd 0.6 x 0.95: 2 0,-1.125; 3 0.95,-1.125; 4 0.95,1.125; 5 0,1.125; 6 -0.95,1.125
JACK2.5_SJ-2523 = smd 2.4 x 2.94: 1 -4.3,-3.274; 2 5.4,-3.424; 3 -1.6,3 | hole 1: -3,0; 3,0

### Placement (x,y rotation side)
C1  29.87,39.69 0 top
C2  40.66,46.67 180 top
C3  33.36,49.53 270 top
C4  40.66,45.4 180 top
C5  34.63,49.53 270 top
C6  35.58,37.78 180 top
C7  36.85,50.16 180 top
C8  36.85,51.75 180 top
C9  11.45,107.95 270 top
C10  61.94,107.95 270 top
C11  29.87,66.99 180 top
C12  60.03,41.27 270 top
C13  52.09,41.27 270 top
C14  31.77,60.64 180 top
C15  35.9,65.4 270 top
C16  37.17,19.37 0 top
C17  33.52,101.12 0 top
C18  43.84,65.56 270 top
C19  49.24,13.02 90 top
C20  30.82,56.51 90 top
C21  57.17,7.62 0 top
C22  39.08,110.17 0 top
C23  39.08,113.19 0 top
CDONE  41.93,35.24 180 top
FID1  2.56,116.84 0 top
FID2  2.56,10.16 0 top
FID3  68.6,10.16 0 top
H1  MHole3.2mm  [MOUNTING_HOLE_1PRIMARY]  6.35,118.87 0 top
H2  MHole3.2mm  [MOUNTING_HOLE_2PRIMARY]  64.26,118.87 0 top
H4  MHole3.2mm  [MOUNTING_HOLE_2PRIMARY]  6.35,6.35 0 top
H301  64.26,6.35 0 top
IC1  56.22,44.77 180 top
IC2  48.28,44.77 180 top
IC3  37.49,101.12 180 top
IC4  31.77,64.13 180 top
IC5  40.03,66.04 270 top
IC6  29.87,52.39 270 top
J1  34.8,10.33 0 top
J2  24.13,114.92 180 top
J3  51.56,115.19 180 top
JP1  61.62,87.63 90 top
JP2  64.16,54.93 270 top
L1  32.73,26.99 0 top
LED1  25.11,51.75 90 top
LED3  25.11,76.52 90 top
LED4  25.11,71.75 90 top
R1  36.06,54.13 90 top
R2  13.36,109.54 90 top
R3  13.36,106.36 90 top
R4  36.54,113.19 90 top
R5  60.03,48.89 90 top
R6  51.46,48.89 90 top
R7  36.54,110.33 270 top
R8  63.84,109.54 90 top
R9  63.84,106.36 90 top
R10  38.44,97.15 270 top
R11  36.54,97.15 270 top
R12  47.65,36.51 270 top
R13  33.36,31.11 270 top
R14  32.25,31.11 270 top
R15  31.42,24.61 0 top
R16  47.33,14.6 270 top
R17  47.33,11.43 270 top
R18  40.35,35.24 90 top
R21  28.92,56.51 90 top
R22  25.11,74.61 180 top
R23  25.11,70.17 180 top
R24  57.17,5.71 180 top
R25  41.62,39.05 0 top
R26  52.57,89.38 270 top
SW1  62.57,64.45 0 top
U1  35.27,43.81 90 top
U2  32.88,21.75 270 top
U3  53.68,73.02 180 top
U4  37.49,106.36 270 top
U$1  [WEEE_BIN_TOP]  12.88,21.27 90 top
U$2  [WEEE_BIN]  15.42,21.27 90 top
U$4  [OSHW_8MM_COPPER]  9.84,63.29 90 top
X2  62.89,74.29 180 top

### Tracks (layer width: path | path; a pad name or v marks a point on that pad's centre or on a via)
!CRESET
  Top 0.254: U1.8 36.02,39.89 36.22,39.69
  Top 0.3: 36.22,39.69 36.54,39.37 40.54,39.37 R25.1 40.85,37.91 41.3,37.46 42.25,37.46 45.11,34.61 58.76,34.61 62.25,38.1 62.25,39.37 62.57,39.69
  Top 0.61: JP2.7 62.57,39.69
!IOB_35B_SPI_SS
  Top 0.254: U1.16 43.89,42.59 46.06,44.77 51.78,44.77 52.73,45.72 57.81,45.72 58.13,46.04 IC1.1
  Top 0.305: IC1.1 R5.1 | JP2.5 58.76,44.77 57.81,45.72
!RAM_CS  (via drill 0.3)
  Top 0.254: v50.19,50.48 IC2.1 | U1.20 42.4,44.59 v44.79,46.99
  Top 0.305: R6.1 50.2,48.13 IC2.1
  Bottom 0.254: v44.79,46.99 46.7,46.99 v50.19,50.48
BOOT_SW
  Top 0.254: 40.35,48.89 38.02,47.68 U1.25
  Top 0.3: SW1.A' SW1.A 57.08,62.45 43.52,48.89 40.35,48.89
CDONE
  Top 0.254: U1.7 35.52,39.75
  Top 0.3: 65.43,42.23 67.02,40.64 67.02,35.24 65.75,33.97 44.47,33.97 42.45,35.99 CDONE.A 41.92,36 R18.2 37.62,38.73 36.22,38.73 35.52,39.44 35.52,39.75
  Top 0.61: JP2.6 65.43,42.23
CLK_12M
  Top 0.3: U1.35 33.02,47.39 arc45 32.83,47.84 arc45 32.58,47.94 31.77,47.94 arc-90 30.67,49.05 30.67,51.43 IC6.3
GND  (via drill 0.3)
  Top 0.3: SW1.B SW1.B' | C6.1 36.85,37.78 v37.17,37.46
  Top 0.4: C13.2 52.22,40.64 v51.14,40.64 | C12.2 v60.03,39.37 | IC1.4 54.24,47.94 v53.36,47.94 | IC2.4 46.3,47.94 v45.43,47.94 | IC3.2 v37.49,103.5 | C17.1 v31.93,101.12
  Top 0.406: R16.1 48.47,15.37 v48.6,15.24 49.24,14.6 C19.2 | R9.1 62.7,105.6 61.94,106.36 C10.2 | R3.1 12.22,105.6 11.45,106.36 C9.2 | 41.77,46.7 C2.1 | R24.2 56.41,7.37 C21.1 | IC4.4 29.9,62.83 v29.87,62.86 | IC4.2 v31.77,64.45 | R22.1 v27.01,74.61 | R23.1 v27.01,70.17
  Top 0.6: R9.1 v63.84,104.14 | R3.1 v13.36,104.46 | C1.1 v28.28,39.69 | v33.36,51.12 C3.1 C5.1 | C20.2 v30.82,58.42 | CDONE.C v41.93,33.34 | v42.57,46.67 41.77,46.7 | C8.1 v38.44,51.75 | C7.1 v38.44,50.16 | U3.2 v53.68,75.56 | C11.2 v27.96,66.99 | C14.2 v29.87,60.64 | C15.2 v35.9,62.86 | IC5.2 v40.03,66.04 | IC5.4 41.33,64.16 v41.3,64.13 | C18.2 v43.84,62.55 | C4.1 C2.1 | R24.2 v55.27,5.71 | U2.2 v32.88,21.75 | C16.2 v39.55,19.37 | X2.1 67.19,80.31 v66.86,80.64 | v56.54,66.52 59.11,66.52 SW1.B | U4.2 v35.27,106.36 | C22.1 v37.81,110.17 | C23.1 v37.81,113.19 | IC6.2 29.16,50.72 v28.92,50.48
  Bottom 0.254: 62.57,46.04 65.75,46.04 | 62.89,43.5 65.75,43.5
  other vias: 35.27,43.81 37.49,43.81 33.04,43.81
  pour Bottom: 69.24,118.82 69.24,6.59 arc-90 64.24,1.59 6.29,1.59 arc-90 1.29,6.59 1.29,118.82 arc-90 6.29,123.82 64.24,123.82 arc-90
IOB_29B_SPI_D3  (via drill 0.3)
  Top 0.254: U1.19 42.69,44.09 v43.04,44.29 | v48.92,43.81 IC2.7
  Top 0.305: IC1.7 56.86,38.73 56.22,38.1 49.55,38.1 48.92,38.73 IC2.7
  Bottom 0.254: v43.04,44.29 48.44,44.29 v48.92,43.81
IOB_31B_SPI_D2  (via drill 0.3)
  Top 0.254: IC2.3 47.65,46.35 47.01,45.72 45.43,45.72 43.3,43.59 U1.18
  Top 0.305: IC1.3 55.59,50.16 v55.27,50.48 | v47.65,50.48 IC2.3
  Bottom 0.305: v55.27,50.48 54,51.75 48.92,51.75 v47.65,50.48
IOB_32A_SPI_SO  (via drill 0.3)
  Top 0.254: U1.14 46.3,41.59 IC2.5
  Top 0.305: IC1.5 54.32,40 v53.68,39.37 | v46.38,39.37 IC2.5
  Bottom 0.305: v46.38,39.37 v53.68,39.37 53.68,45.08 60.98,52.39 JP2.2
IOB_33B_SPI_SI
  Top 0.254: U1.17 43.59,43.09 45.74,45.24 48.12,45.24 48.92,46.04 IC2.2
  Top 0.305: IC2.2 48.92,50.8 49.87,51.75 55.9,51.75 56.86,50.8 | 56.86,50.8 IC1.2 | 56.86,50.8 61.3,50.8 62.25,49.85 JP2.3
IOB_34A_SPI_SCK  (via drill 0.3)
  Top 0.254: U1.15 44.34,42.09 46.06,43.81 47.33,43.81 47.65,43.5 IC2.6
  Top 0.305: IC1.6 55.59,39.37 v54.95,38.73 | IC2.6 v47.65,38.73 R12.1
  Bottom 0.305: v47.65,38.73 v54.95,38.73 54.95,44.45 57.81,47.31 JP2.4
N$1
  Top 0.3: U1.40 30.65,45.09 29.71,46.04 27.65,46.04 25.11,48.58 LED1.2
N$2
  Top 0.3: U3.6 55.73,71.9 56.22,72.39 56.22,76.45 X2.2
N$3
  Top 0.3: R7.2 36.54,107.53 U4.1
N$3_N
  Top 0.7: J2.2 25.57,110.21 26.69,111.33 36.54,111.33 | 36.54,111.33 41.76,111.33 44.3,108.79 50.05,108.79 52.56,111.31 J3.2 | R7.1 36.54,111.33
N$3_P
  Top 0.406: R4.1 36.46,112.43 36.22,112.19
  Top 0.7: J2.3 26.67,112.21 26.69,112.19 36.22,112.19 42.11,112.19 44.65,109.65 49.69,109.65 50.52,110.47 50.52,112.45 J3.3
N$4
  Top 0.406: R24.1 57.94,7.37 C21.2
  Top 0.7: H301.B3,2 58.57,6.35 R24.1
N$5
  Top 0.3: LED3.C 24.36,74.62 R22.2
N$6
  Top 0.3: R2.1 R3.2
N$7
  Top 0.3: R8.1 R9.2
N$8  (via drill 0.3)
  Top 0.3: R4.2 38.79,113.95 v39.08,113.98 | U4.6 38.61,109.05 v38.6,109.06
  Bottom 0.3: v39.08,113.98 39.08,109.54 v38.6,109.06
N$9
  Top 0.3: R8.2 62.7,110.3 61.94,109.54 C10.1
  Top 0.61: J3.P$1 61.36,115.19 63.84,112.71 R8.2
  Bottom 0.61: J3.P$2 J3.P$1
N$10
  Top 0.3: IC3.1 38.44,105.24 U4.4
N$11
  Top 0.3: C9.1 11.45,109.54 12.09,110.17 13.23,110.17 R2.2
  Top 0.61: J2.Z2 15.89,114.92 13.36,112.39 R2.2
  Bottom 0.61: J2.Z2 J2.Z1
N$12
  Top 0.3: 36.54,97.98 R11.1
  Top 0.305: IC3.4 36.54,97.98
N$13
  Top 0.3: 38.44,97.98 R10.1
  Top 0.305: IC3.6 38.44,97.98
N$14
  Top 0.3: R23.2 LED4.C
N$15
  Top 0.3: IC3.3 36.54,105.24 U4.3
N$17_D_N
  Top 0.254: L1.3 33.15,27.84
  Top 0.406: 33.15,30.16 33.36,30.16 R13.2
  Top 0.7: 33.15,27.84 33.15,30.16
N$17_D_P
  Top 0.4: L1.2 32.3,27.84
  Top 0.406: 32.3,30.16 32.25,30.16 R14.2
  Top 0.7: 32.3,27.84 32.3,30.16
N$25
  Top 0.3: R21.1 29.07,55.6 29.07,54.77 29.23,54.61 29.23,53.32 IC6.1
N$45
  Top 0.3: LED1.1 24.11,48.62 27.33,45.4 29.23,45.4 30.04,44.59 U1.41
N$52
  Top 0.3: C7.2 36.09,48.77 36.02,48.69 U1.29
  Top 0.406: C7.2 C8.2 36.09,53.34 R1.1
N$55
  Top 0.406: R17.1 R16.2
N$61
  Top 0.406: J1.Z2 47,10.33 R17.2 48.47,10.67 49.24,11.43 C19.1
  Top 0.813: J1.Z1 J1.Z2
N$63
  Top 0.3: U1.39 31.26,45.59 30.03,46.83 27.96,46.83 26.11,48.69 LED1.3
RX
  Top 0.254: U1.26 37.52,48.29 38.28,48.74 38.92,48.74 40.66,50.48
  Top 0.3: 40.66,50.48 52.73,62.55 U3.4
TAP_D_N
  Top 0.3: U1.43 31.24,43.59 30.82,43.5 25.11,43.5 20.82,47.78 20.82,76.68 36.54,92.39 R11.2
TAP_D_P
  Top 0.3: U1.42 25.46,44.09 21.52,48.04 21.52,76.42 37.81,92.71 38.44,93.32 R10.2
TX
  Top 0.254: U1.27 37.02,48.42 37.81,49.21 38.76,49.21 40.03,50.48
  Top 0.3: 40.03,50.48 40.03,51.12 51.46,62.55 51.46,72.88 U3.3
UART_TX0
  Top 0.3: U3.1 54.63,79.37 56.22,80.96 60.03,80.96 63.21,77.79 63.21,73.02 63.84,72.39 63.84,71.94 X2.3
USB0_D_N
  Top 0.7: U2.4 33.81,20.8 31.88,18.87 31.88,14.78 32.27,14.4 33.36,14.4 33.36,14.85 J1.2
USB0_D_P
  Top 0.7: U2.3 31.76,20.02 31.79,19.99 31.03,19.23 31.03,14.43 31.91,13.54 33.36,13.54 33.36,13.24 J1.3
USB1_D_N
  Top 0.4: 33.15,26.03 33.15,26.11 L1.4
  Top 0.7: U2.6 33.63,22.7 33.15,23.18 33.15,26.03
USB1_D_P
  Top 0.3: R15.2 32.22,25 32.3,25.08
  Top 0.406: 32.3,26.03 32.3,26.11 L1.1
  Top 0.7: U2.1 31.82,22.7 32.3,23.18 32.3,25.08 32.3,26.03
USB_D_N
  Top 0.3: U1.4 34.02,39.31
  Top 0.4: 33.66,38.43 33.56,38.54
  Top 0.406: 34.02,39.31 33.84,38.73 arc-89 33.56,38.54 | 33.15,32.07 33.15,31.83 R13.1
  Top 0.7: 33.66,38.43 33.15,37.92 33.15,32.07
USB_D_P
  Top 0.3: U1.3 33.52,39.53 | 33.52,39.53 | 33.06,39.04 33.16,38.93 33.52,39.53
  Top 0.406: 32.3,32.07 32.3,31.67 R14.1
  Top 0.7: 33.06,39.04 32.3,38.28 32.3,32.07
USB_DET
  Top 0.254: U1.2 33.02,39.98 32.25,39.37
  Top 0.3: 32.25,39.37 30.69,37.97 30.69,24.64 R15.1
VBUS_DUT
  Top 0.6: U4.5 53.16,106.36 55.06,108.27 | R26.1 57.46,90.14 57.49,90.17 JP1.3
  Top 0.813: J3.1 55.06,108.27 55.06,108.16 59.08,104.14 JP1.3
  Top 1: J2.1 21.57,110.21 20.66,111.12 20.66,113.03 26.06,118.43 50.19,118.43 55.06,113.55 J3.1
VBUS_HOST  (via drill 0.3)
  Top 0.6: 36.05,20.8 35.11,21.75 U2.5 | C16.1 36.05,19.37
  Top 0.813: v67.33,85.09 JP1.1
  Top 1: J1.1 v36.05,17.46 36.05,19.37 36.05,20.8
  Bottom 0.813: v36.05,17.46 58.13,17.46 68.29,27.62 68.29,84.14 v67.33,85.09
VCC_1V2  (via drill 0.3)
  Top 0.185: 35.52,47.56 35.49,47.56 35.42,47.62
  Top 0.254: U1.5 34.52,38.11
  Top 0.3: U1.30 35.52,47.56 | 35.42,47.62 35.11,47.94 34.95,47.94 34.63,48.26 C5.2 34.82,48.77 v35.42,49.37 | IC5.3 38.73,62.83 37.81,61.91 35.33,61.91 33.87,60.45 | C6.2 34.82,37.81 34.52,38.11
  Top 0.4: R1.2 36.06,56.67 v35.9,56.83 35.9,58.42 33.87,60.45 33.04,60.45 | v34.95,36.83 34.95,37.66 C6.2
  Top 0.406: IC4.5 32.72,60.77 | 32.72,60.77 33.04,60.45 | C14.1 32.59,60.64 32.72,60.77
  Bottom 0.3: v35.9,56.83 35.42,56.36 v35.42,49.37 35.42,47.15 34.31,46.04 34.31,41.91 34.95,41.27 v34.95,36.83
VCC_3V3  (via drill 0.3)
  Top 0.254: 61.62,48.58 65.75,48.58 | U1.24 39.63,46.59 39.71,46.67 | 62.25,43.5 66.06,43.5 | 62.25,46.04 66.06,46.04
  Top 0.3: C3.2 33.38,48.75 33.38,48.24 34.02,47.6 U1.33 | U1.24 39.66,46.59 C2.2 | 30.67,55.6 C20.1 | C4.2 39.23,45.4 39.04,45.59 U1.22 | U1.1 32.52,40.27 31.77,39.69
  Top 0.4: IC1.8 58.37,41.52 58.76,41.91 59.9,41.91 C12.1 | IC2.8 50.43,41.52 50.95,42.04 C13.1 52.09,43.5 v51.78,43.81 | C17.2 37.01,101.12 37.49,100.65 IC3.5 | R5.2 60.54,49.66 61.62,48.58 | C1.2 31.77,39.69
  Top 0.406: R12.2 46.89,35.75 46.7,35.56 | IC6.4 30.56,54.35 30.82,54.61 C20.1
  Top 0.6: C4.2 C2.2 | IC5.5 43.81,66.99 C18.1
  Bottom 0.4: v51.78,43.81 v51.78,46.67
  Bottom 0.6: v34,58.74 v37.17,58.74
  pour Top: 69.24,118.82 69.24,6.59 arc-90 64.24,1.59 6.29,1.59 arc-90 1.29,6.59 1.29,118.82 arc-90 6.29,123.82 64.24,123.82 arc-90
VIN
  Top 0.406: LED4.A 27.01,71.75 30.5,68.26 30.5,66.67 30.82,66.67
  Top 0.6: IC5.1 36.09,66.99 C15.1 35.77,66.67 32.73,66.67 | 53.05,87.63 32.73,67.31 32.73,66.67 | IC4.3 30.82,66.8 C11.1 | 32.73,66.67 30.95,66.67 C11.1 | IC4.1 32.72,66.67 32.73,66.67 | 30.82,66.67 30.82,66.8 C11.1 | 53.05,87.63 JP1.2 | R26.2 52.57,88.11 53.05,87.63

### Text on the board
Top: iCE40-usbtrace v | (C) 2022 sysmocom GmbH | CC-BY-SA 3.0
tNames: VBUS_DUT | VBUS_HOST | supply by | 3V3 | iCE40-usbtrace v | (C) 2022 sysmocom GmbH | CC-BY-SA 3.0 | VIN | 3V3 | SI | SO | SCK | SS | CDO | CRE | GND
